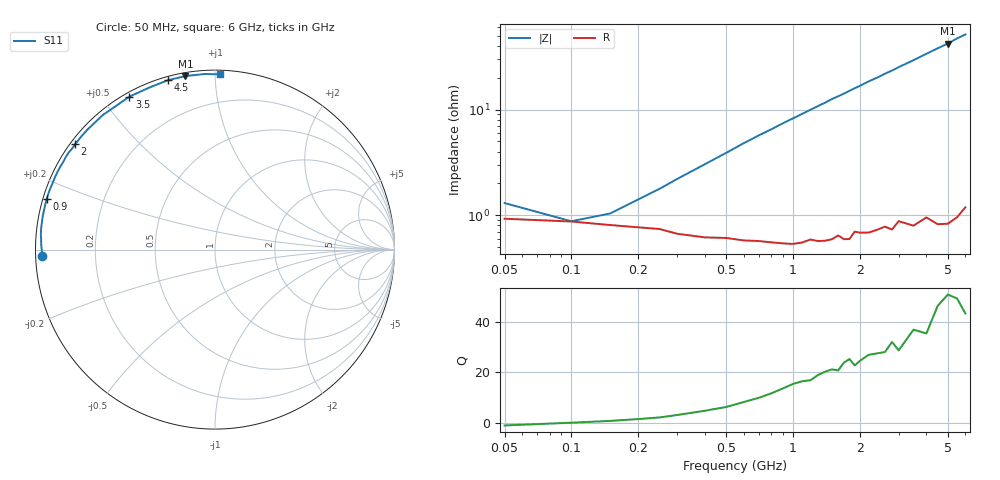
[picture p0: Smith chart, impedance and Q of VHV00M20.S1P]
! Infineon Technologies  Discrete & RF Semiconductors
! BB 814
! Si Tuning Diode in SOT23
! VR =
! S-Parameters:  July  1999
# GHz  S  MA  R  50
!  f  S11
! GHz  MAG  ANG
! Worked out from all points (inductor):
!   34 points, 50 MHz to 6 GHz, reference 50 ohm
!   read as one part to ground: L = 1.18 nH near 300 MHz
!   highest Q = 49.3 at 5 GHz (marker M1), where L = 1.34 nH
!   S11 on the Smith chart (normalised r, x): 50 MHz: 0.02, -0.02; 900 MHz: 0.01, +0.15; 2 GHz: 0.01, +0.33; 3.5 GHz: 0.02, +0.59; 4.5 GHz: 0.02, +0.76; 6 GHz: 0.02, +1.03
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0.05  0.9637 -177.9
0.1  0.9658 179.8
0.2  0.9698 177.3
0.3  0.9737 175.2
0.4  0.9757 173.2
0.6  0.9774 169.1
0.8  0.9785 165.2
0.9  0.9791 163.2
1.1  0.9789 159.4
1.3  0.9785 155.6
1.4  0.9785 153.8
1.5  0.978 151.8
1.6  0.9763 150.1
1.7  0.9783 148.4
1.8  0.9784 146.5
1.9  0.9749 144.7
2  0.9757 143.0
2.2  0.9762 139.4
2.4  0.9752 136.3
2.6  0.9742 132.8
2.8  0.9763 129.8
3  0.9724 126.5
3.5  0.9766 119.2
4  0.9742 112.0
4.5  0.9794 105.5
5  0.9808 99.7
5.5  0.9799 93.4
6  0.9772 88.4
